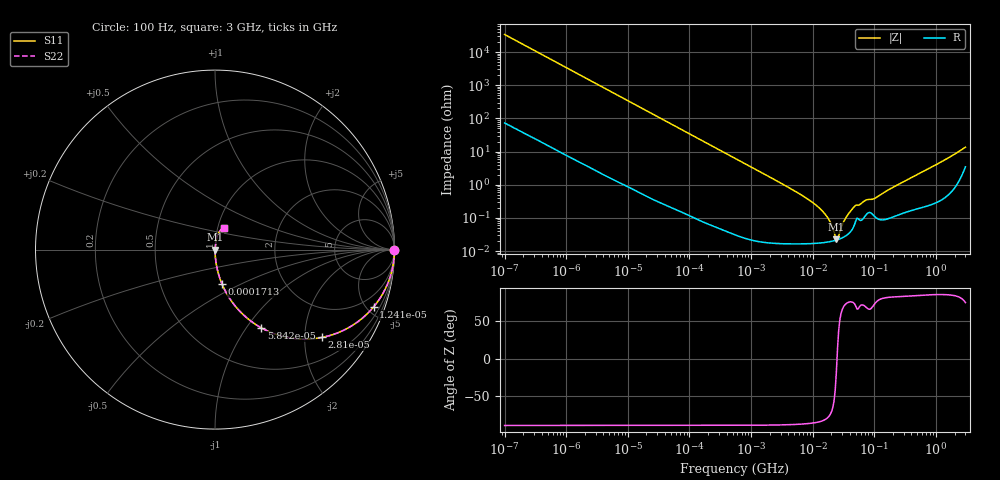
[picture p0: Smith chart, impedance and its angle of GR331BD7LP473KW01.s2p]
!Murata Part Number: GR331BD7LP473KW01
!These Parameters are Measured in Series Mode Connection
!Data Generated on Jun 10, 2025
!  o--ll--o
!Port1  Port2
!  o------o
!Operation Temp=25[degC], DC Bias Voltage=0[V]
!Freq. Start=100[Hz] Stop=3[GHz] 401[Steps]
# Hz S RI R 50
!Freq.(Hz) S11(Real) S11(Imag) S21(Real) S21(Imag) S12(Real) S12(Imag) S22(Real) S22(Imag)
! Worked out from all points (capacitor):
!   401 points, 100 Hz to 3 GHz, reference 50 ohm
!   read as one part in series: C = 46.8 nF near 109 Hz
!   lowest |Z| = 22.6 mohm at 24.18 MHz (marker M1)
!   series resonance near 24.79 MHz, so ESL is about 880 pH
!   S11 on the Smith chart (normalised r, x): 100 Hz: open; 12.4 kHz: 1.01, -5.52; 28.1 kHz: 1.01, -2.44; 58.42 kHz: 1.00, -1.17; 171.3 kHz: 1.00, -0.40; 3 GHz: 1.07, +0.26
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100  1 -0.00294  1.5e-05 0.00294  1.5e-05 0.00294  1 -0.00294
1788  0.9971 -0.0523  0.00286 0.0523  0.00286 0.0523  0.9971 -0.0523
5024  0.9785 -0.1438  0.0215 0.1438  0.0215 0.1438  0.9785 -0.1438
12405  0.8832 -0.3199  0.1168 0.3199  0.1168 0.3199  0.8832 -0.3199
28103  0.5974 -0.4891  0.4026 0.4891  0.4026 0.4891  0.5974 -0.4891
31977  0.5344 -0.4974  0.4656 0.4974  0.4656 0.4974  0.5344 -0.4974
58416  0.257 -0.4354  0.743 0.4354  0.743 0.4354  0.257 -0.4354
93790  0.119 -0.3221  0.881 0.3221  0.881 0.3221  0.119 -0.3221
171338  0.0393 -0.1926  0.9607 0.1926  0.9607 0.1926  0.0393 -0.1926
547723  0.00424 -0.0626  0.9958 0.0626  0.9958 0.0626  0.00424 -0.0626
4141163  0.00023 -0.0081  0.9998 0.0081  0.9998 0.0081  0.00023 -0.0081
9794414  0.000178 -0.00298  0.9998 0.00298  0.9998 0.00298  0.000178 -0.00298
1.641694e7  0.000185 -0.00119  0.9998 0.00119  0.9998 0.00119  0.000185 -0.00119
1.950129e7  0.000195 -0.00068  0.9998 0.00068  0.9998 0.00068  0.000195 -0.00068
2.418395e7  0.000215 -6.93e-05  0.9998 6.93e-05  0.9998 6.93e-05  0.000215 -6.93e-05
2.635803e7  0.000226 0.000175  0.9998 -0.000175  0.9998 -0.000175  0.000226 0.000175
3.412477e7  0.000286 0.000938  0.9997 -0.000938  0.9997 -0.000938  0.000286 0.000938
4.612319e7  0.000548 0.00201  0.9995 -0.00201  0.9995 -0.00201  0.000548 0.00201
7.405258e7  0.00127 0.00323  0.9987 -0.00323  0.9987 -0.00323  0.00127 0.00323
1.044919e8  0.00106 0.00387  0.9989 -0.00387  0.9989 -0.00387  0.00106 0.00387
1.751444e8  0.00102 0.0072  0.999 -0.0072  0.999 -0.0072  0.00102 0.0072
3e9  0.0487 0.1204  0.9513 -0.1204  0.9513 -0.1204  0.0487 0.1204
